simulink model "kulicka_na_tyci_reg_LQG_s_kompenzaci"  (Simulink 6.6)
settings: Solver=ode45  StartTime=0.0  StopTime=inf  FixedStep=0.01  RelTol=1e-3
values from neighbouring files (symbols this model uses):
  K = tf(num,den)    [phinf2.m]
  Ng = lqr_kompenzace(A,B,C,D,K)    [kulicka_na_tyci_LQG_podklad.m]    (also in lqr_kompenzace.m = Nu + K*Nx; testx.m; kockaLQG.m; kockaLQR.m)
  Ts = 0.02    [kulicka_na_tyci_LQG_podklad.m]    (also in podklad.m = 0.1; nadoby.m = 0.1; nadoby_prediktivni.m = 0.0005)
undefined symbols (not defined in the file or in its folder): Humusoft, Kalmf, MF624, to, V
libraries: rtlib x4, simulink x1

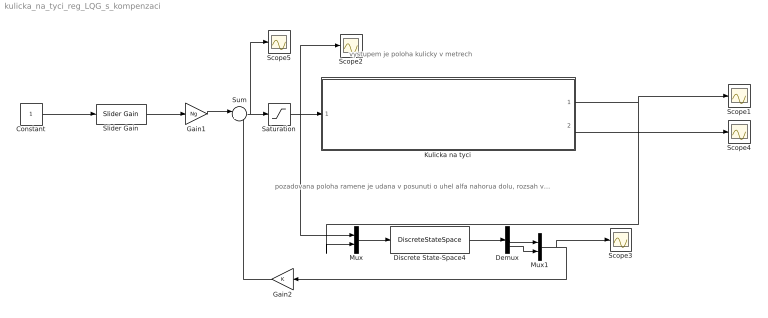
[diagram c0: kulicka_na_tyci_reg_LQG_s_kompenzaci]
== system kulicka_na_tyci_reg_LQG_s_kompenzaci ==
  note: pozadovana poloha ramene je udana v posunuti o uhel alfa nahorua dolu, rozsah vstupu do soustavy je: [-0.01 ; 0.01] , kde 0 je nulova odchylka ramene
  note: vystupem je poloha kulicky v metrech
  Constant : Constant
  Demux : Demux  Outputs=3
  Discrete State-Space4 : DiscreteStateSpace  A=Kalmf.a  B=Kalmf.b  C=Kalmf.c  D=Kalmf.d  SampleTime=Ts
  Gain1 : Gain  Gain=Ng
  Gain2 : Gain  Orientation=left  Gain=K  Multiplication=Matrix(K*u)
  Kulicka na tyci : Subsystem  TreatAsAtomicUnit=on  mask{Ts=0.01, IN_K=1, IN_R=2, OUT_S=1}
      mask prompts: Ts "Vzorkovaci perioda [s]"; IN_K "Cislo analog. vstupu - poloha kulicky"; IN_R "Cislo analog. vstupu - poloha ramane"; OUT_S "Cislo analog vystutpu - rizeni naklonu"
  Mux : Mux  Inputs=2
  Mux1 : Mux  Inputs=2
  Saturation : Saturate  UpperLimit=0.01  LowerLimit=-0.01  ZeroCross=off  SampleTime=0.01
  Scope{1..5} (5 alike) : Scope
  Slider Gain : simulink/Math Operations/Slider Gain  SystemSampleTime=-1  low=0  gain=0.33  high=1
  Sum : Sum  Inputs=|+-
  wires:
  Kulicka na tyci/1(kulicka) -> Scope1/1, Mux/2
  Constant/1 -> Slider Gain/1
  Mux/1 -> Discrete State-Space4/1
  Discrete State-Space4/1 -> Demux/1
  Demux/3 -> Mux1/2
  Demux/2 -> Mux1/1
  Mux1/1 -> Gain2/1, Scope3/1
  Gain2/1 -> Sum/2
  Sum/1 -> Saturation/1, Scope5/1
  Saturation/1 -> Kulicka na tyci/1(rameno), Mux/1, Scope2/1
  Kulicka na tyci/2(rameno out) -> Scope4/1
  Slider Gain/1 -> Gain1/1
  Gain1/1 -> Sum/1

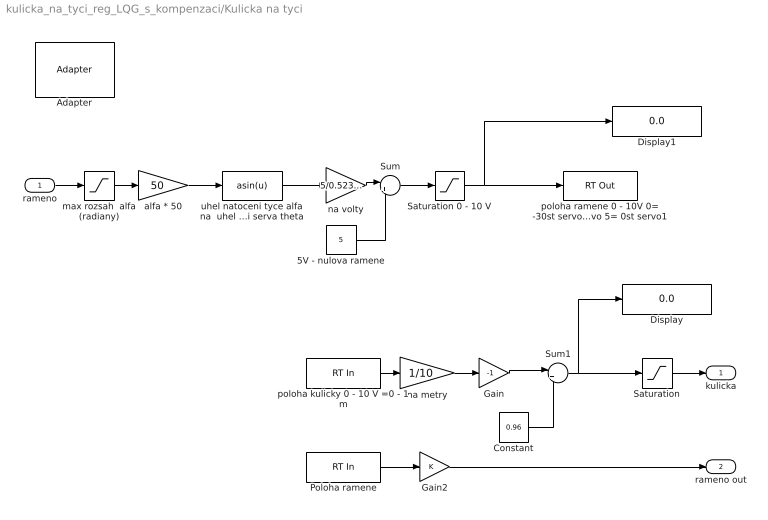
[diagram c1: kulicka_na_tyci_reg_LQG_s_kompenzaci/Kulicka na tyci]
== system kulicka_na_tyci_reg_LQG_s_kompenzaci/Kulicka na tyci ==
  rameno : Inport
  5V - nulova ramene : Constant  Value=5
  Adapter : rtlib/Adapter  SystemSampleTime=-1  DriverName=Humusoft/MF624  DriverAddress=4294967295  DriverOptions=0
  Constant : Constant  Value=0.96
  Display : Display
  Display1 : Display
  Gain : Gain  Gain=-1
  Gain2 : Gain
  Poloha ramene : rtlib/RT In  SampleTime=Ts  Adapter=Adapter  IOClass=Analog Input  Channels=IN_R  SLDataType=double  MaxMissedTicks=100  ShowMissedTicks=off  YieldWhenWaiting=on  AIORange=-10 to 10 V  AIOUnits=Volts  DIOMode=Bit  CIReset=never  CIEdge=rising  CIGate=none  EIQuadrature=quadruple  EIIndexPulse=reset  EIFilterFrequency=Inf  OIOParameters=[]
  Saturation : Saturate  UpperLimit=0.95  LowerLimit=0  ZeroCross=off
  Saturation 0 - 10 V : Saturate  UpperLimit=10  LowerLimit=0  ZeroCross=off
  Sum : Sum  Inputs=|++
  Sum1 : Sum  Inputs=|++
  alfa * 50 : Gain  Gain=50
  max rozsah  alfa (radiany) : Saturate  UpperLimit=0.01  LowerLimit=-0.01  ZeroCross=off
  na metry : Gain  Gain=1/10
  na volty : Gain  Gain=5/0.52359877559830
  poloha kulicky 0 - 10 V =0 - 1 m : rtlib/RT In  SampleTime=Ts  Adapter=Adapter  IOClass=Analog Input  Channels=IN_K  SLDataType=double  MaxMissedTicks=100  ShowMissedTicks=off  YieldWhenWaiting=on  AIORange=-10 to 10 V  AIOUnits=Volts  DIOMode=Bit  CIReset=never  CIEdge=rising  CIGate=none  EIQuadrature=quadruple  EIIndexPulse=reset  EIFilterFrequency=Inf  OIOParameters=[]
  poloha ramene 0 - 10V 0= -30st servo 10= +30st servo 5= 0st servo1 : rtlib/RT Out  SampleTime=Ts  Adapter=Adapter  IOClass=Analog Output  Channels=OUT_S  InitialValue=[0]  FinalValue=[0]  MaxMissedTicks=100  ShowMissedTicks=off  YieldWhenWaiting=on  AIORange=-10 to 10 V  AIOUnits=Volts  DIOMode=Bit  OIOParameters=[]
  uhel natoceni tyce alfa na  uhel natoceni serva theta : Fcn  Expr=asin(u)
  kulicka : Outport
  rameno out : Outport  Port=2
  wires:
  poloha kulicky 0 - 10 V =0 - 1 m/1 -> na metry/1
  rameno/1 -> max rozsah  alfa (radiany)/1
  Saturation 0 - 10 V/1 -> Display1/1, poloha ramene 0 - 10V 0= -30st servo 10= +30st servo 5= 0st servo1/1
  Poloha ramene/1 -> Gain2/1
  Gain2/1 -> rameno out/1
  uhel natoceni tyce alfa na  uhel natoceni serva theta/1 -> na volty/1
  alfa * 50/1 -> uhel natoceni tyce alfa na  uhel natoceni serva theta/1
  max rozsah  alfa (radiany)/1 -> alfa * 50/1
  na volty/1 -> Sum/1
  5V - nulova ramene/1 -> Sum/2
  Sum/1 -> Saturation 0 - 10 V/1
  na metry/1 -> Gain/1
  Saturation/1 -> kulicka/1
  Gain/1 -> Sum1/1
  Sum1/1 -> Saturation/1, Display/1
  Constant/1 -> Sum1/2
